FUNCTION FC 117 : VOID
TITLE =BLOCK INLETS 1 AND 2 - FRONT AND REAR
AUTHOR : Esposito
FAMILY : EGAL_srl
NAME : INLET_P
VERSION : 0.1

BEGIN
NETWORK
TITLE =CONDITIONS FOR ENABLE INLETS
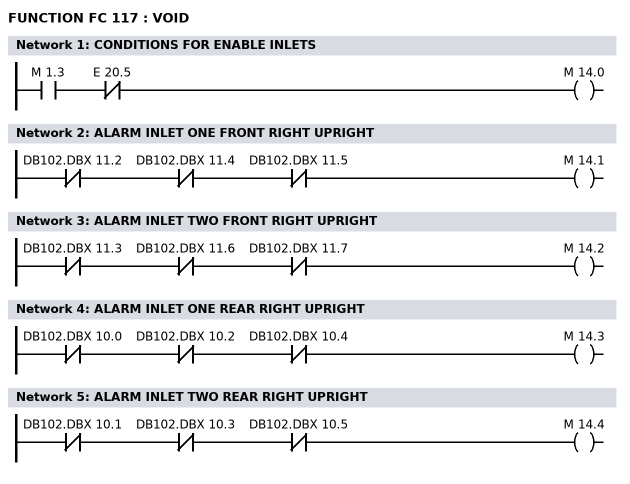
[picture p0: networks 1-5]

      U     M      1.3;
      UN    E     20.5;
      =     M     14.0;
NETWORK
TITLE =ALARM INLET ONE FRONT RIGHT UPRIGHT

      UN    DB102.DBX   11.2;
      UN    DB102.DBX   11.4;
      UN    DB102.DBX   11.5;
      =     M     14.1;
NETWORK
TITLE =ALARM INLET TWO FRONT RIGHT UPRIGHT

      UN    DB102.DBX   11.3;
      UN    DB102.DBX   11.6;
      UN    DB102.DBX   11.7;
      =     M     14.2;
NETWORK
TITLE =ALARM INLET ONE REAR RIGHT UPRIGHT

      UN    DB102.DBX   10.0;
      UN    DB102.DBX   10.2;
      UN    DB102.DBX   10.4;
      =     M     14.3;
NETWORK
TITLE =ALARM INLET TWO REAR RIGHT UPRIGHT

      UN    DB102.DBX   10.1;
      UN    DB102.DBX   10.3;
      UN    DB102.DBX   10.5;
      =     M     14.4;
NETWORK
TITLE =LOAD VALUE TIME INLET ONE FRONT RIGHT UPRIGHT

      L     DB15.DBW  180;
      ITB   ;
      L     W#16#2000; // Base times one seconds
      OW    ;
      T     LW   100; // word of register temporary
NETWORK
TITLE =START/STOP INLET ONE FRONT RIGHT UPRIGHT
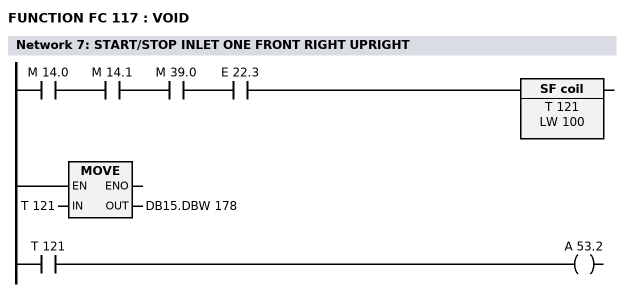
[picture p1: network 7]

      U     M     14.0;
      U     M     14.1;
      U     M     39.0;
      U     E     22.3;
      L     LW   100;
      SA    T    121;
      NOP   0;
      L     T    121;
      T     DB15.DBW  178;
      NOP   0;
      U     T    121;
      =     A     53.2;
NETWORK
TITLE =LOAD VALUE TIME INLET TWO FRONT RIGHT UPRIGHT

      L     DB15.DBW  184;
      ITB   ;
      L     W#16#2000;
      OW    ;
      T     LW   104;
NETWORK
TITLE =START/STOP INLET TWO FRONT RIGHT UPRIGHT
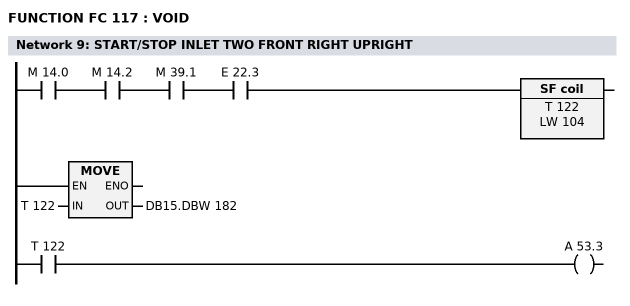
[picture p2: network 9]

      U     M     14.0;
      U     M     14.2;
      U     M     39.1;
      U     E     22.3;
      L     LW   104;
      SA    T    122;
      NOP   0;
      L     T    122;
      T     DB15.DBW  182;
      NOP   0;
      U     T    122;
      =     A     53.3;
NETWORK
TITLE =LOAD VALUE TIME INLET ONE REAR RIGHT

      L     DB15.DBW  188;
      ITB   ;
      L     W#16#2000;
      OW    ;
      T     LW   108;
NETWORK
TITLE =START/STOP INLET ONE REAR RIGHT UPRIGHT
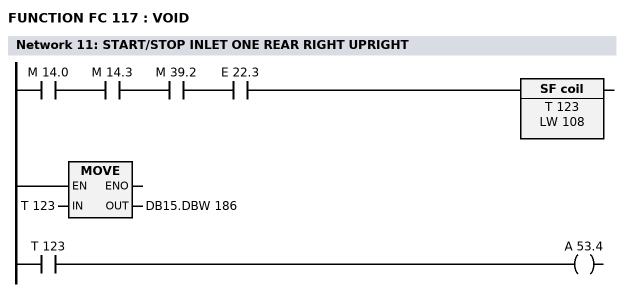
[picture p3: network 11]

      U     M     14.0;
      U     M     14.3;
      U     M     39.2;
      U     E     22.3;
      L     LW   108;
      SA    T    123;
      NOP   0;
      L     T    123;
      T     DB15.DBW  186;
      NOP   0;
      U     T    123;
      =     A     53.4;
NETWORK
TITLE =LOAD VALUE TIME INLET TWO REAR RIGHT UPRIGHT

      L     DB15.DBW  192;
      ITB   ;
      L     W#16#2000;
      OW    ;
      T     LW   112;
NETWORK
TITLE =START/STOP INLET TWO REAR RIGHT UPRIGHT
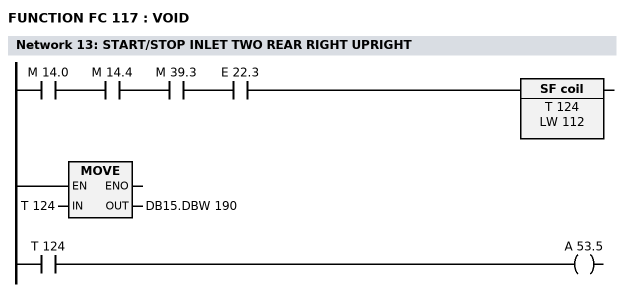
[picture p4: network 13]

      U     M     14.0;
      U     M     14.4;
      U     M     39.3;
      U     E     22.3;
      L     LW   112;
      SA    T    124;
      NOP   0;
      L     T    124;
      T     DB15.DBW  190;
      NOP   0;
      U     T    124;
      =     A     53.5;
END_FUNCTION

